DATA_BLOCK "Telegramindeling_rcv"
TITLE =
AUTHOR : DSB_TIM
FAMILY : Tim_rcv
NAME : Receive
VERSION : 0.1


  STRUCT
 Telegram101  :  STRUCT
besturing_remote  : BOOL ;
besturing_lokaal  : BOOL ;
pompen_blokkering  : BOOL ;
pompen_vrijgeven  : BOOL ;
niveaumeting1_voorkeuze  : BOOL ;
niveaumeting2_voorkeuze  : BOOL ;
regenpompen_blokkering  : BOOL ;
regenpompen_vrijgeven  : BOOL ;
END_STRUCT;
Telegram102  :  STRUCT
besturing_remote  : BOOL ;
besturing_lokaal  : BOOL ;
pompen_blokkering  : BOOL ;
pompen_vrijgeven  : BOOL ;
niveaumeting1_voorkeuze  : BOOL ;
niveaumeting2_voorkeuze  : BOOL ;
regenpompen_blokkering  : BOOL ;
regenpompen_vrijgeven  : BOOL ;
END_STRUCT;
Telegram103  :  STRUCT
besturing_remote  : BOOL ;
besturing_lokaal  : BOOL ;
pompen_blokkering  : BOOL ;
pompen_vrijgeven  : BOOL ;
niveaumeting1_voorkeuze  : BOOL ;
niveaumeting2_voorkeuze  : BOOL ;
regenpompen_blokkering  : BOOL ;
regenpompen_vrijgeven  : BOOL ;
END_STRUCT;
Telegram104  :  STRUCT
besturing_remote  : BOOL ;
besturing_lokaal  : BOOL ;
pompen_blokkering  : BOOL ;
pompen_vrijgeven  : BOOL ;
niveaumeting1_voorkeuze  : BOOL ;
niveaumeting2_voorkeuze  : BOOL ;
regenpompen_blokkering  : BOOL ;
regenpompen_vrijgeven  : BOOL ;
END_STRUCT;
Telegram105  :  STRUCT
besturing_remote  : BOOL ;
besturing_lokaal  : BOOL ;
pompen_blokkering  : BOOL ;
pompen_vrijgeven  : BOOL ;
niveaumeting1_voorkeuze  : BOOL ;
niveaumeting2_voorkeuze  : BOOL ;
regenpompen_blokkering  : BOOL ;
regenpompen_vrijgeven  : BOOL ;
END_STRUCT;
Telegram106  :  STRUCT
besturing_remote  : BOOL ;
besturing_lokaal  : BOOL ;
pompen_blokkering  : BOOL ;
pompen_vrijgeven  : BOOL ;
niveaumeting1_voorkeuze  : BOOL ;
niveaumeting2_voorkeuze  : BOOL ;
regenpompen_blokkering  : BOOL ;
regenpompen_vrijgeven  : BOOL ;
END_STRUCT;

Telegram140  :  STRUCT
reserve1  : WORD ;
END_STRUCT;
Telegram141  :  STRUCT
reserve2  : WORD ;
END_STRUCT;
Telegram142  :  STRUCT
reserve3  : WORD ;
END_STRUCT;
Telegram143  :  STRUCT
reserve4  : WORD ;
END_STRUCT;
Telegram144  :  STRUCT
reserve5  : WORD ;
END_STRUCT;
Telegram145  :  STRUCT
reserve6  : WORD ;
END_STRUCT;
Telegram146  :  STRUCT
laagwater  : WORD ;
END_STRUCT;
Telegram147  :  STRUCT
laagwater_herstel  : WORD ;
END_STRUCT;
Telegram148  :  STRUCT
hoogwater  : WORD ;
END_STRUCT;
Telegram149  :  STRUCT
hoogwater_herstel  : WORD ;
END_STRUCT;
Telegram150  :  STRUCT
dode_band_niveaumeting  : WORD ;
END_STRUCT;
Telegram151  :  STRUCT
reserve7  : WORD ;
END_STRUCT;
Telegram152  :  STRUCT
dode_band_logging  : WORD ;
END_STRUCT;
Telegram153  :  STRUCT
pomp_1_inslagpeil  : WORD ;
END_STRUCT;
Telegram154  :  STRUCT
pomp_2_inslagpeil  : WORD ;
END_STRUCT;
Telegram155  :  STRUCT
pomp_3_inslagpeil  : WORD ;
END_STRUCT;
Telegram156  :  STRUCT
pomp_4_inslagpeil  : WORD ;
END_STRUCT;
Telegram157  :  STRUCT
pomp_5_inslagpeil  : WORD ;
END_STRUCT;
Telegram158  :  STRUCT
pomp_6_inslagpeil  : WORD ;
END_STRUCT;
Telegram159  :  STRUCT
pomp_1_uitslagpeil  : WORD ;
END_STRUCT;
Telegram160  :  STRUCT
pomp_2_uitslagpeil  : WORD ;
END_STRUCT;
Telegram161  :  STRUCT
pomp_3_uitslagpeil  : WORD ;
END_STRUCT;
Telegram162  :  STRUCT
pomp_4_uitslagpeil  : WORD ;
END_STRUCT;
Telegram163  :  STRUCT
pomp_5_uitslagpeil  : WORD ;
END_STRUCT;
Telegram164  :  STRUCT
pomp_6_uitslagpeil  : WORD ;
END_STRUCT;
Telegram165  :  STRUCT
reserve8  : WORD ;
END_STRUCT;
Telegram166  :  STRUCT
reserve9  : WORD ;
END_STRUCT;
Telegram167  :  STRUCT
reserve10  : WORD ;
END_STRUCT;
Telegram168  :  STRUCT
reserve11  : WORD ;
END_STRUCT;
Telegram169  :  STRUCT
reserve12  : WORD ;
END_STRUCT;
Telegram170  :  STRUCT
reserve13  : WORD ;
END_STRUCT;
Telegram171  :  STRUCT
reserve14  : WORD ;
END_STRUCT;
Telegram172  :  STRUCT
reserve15  : WORD ;
END_STRUCT;


  END_STRUCT ;
BEGIN

Telegram101.besturing_remote   := FALSE;
Telegram101.besturing_lokaal   := FALSE;
Telegram101.pompen_blokkering   := FALSE;
Telegram101.pompen_vrijgeven   := FALSE;
Telegram101.niveaumeting1_voorkeuze   := FALSE;
Telegram101.niveaumeting2_voorkeuze   := FALSE;
Telegram101.regenpompen_blokkering   := FALSE;
Telegram101.regenpompen_vrijgeven   := FALSE;


Telegram102.besturing_remote   := FALSE;
Telegram102.besturing_lokaal   := FALSE;
Telegram102.pompen_blokkering   := FALSE;
Telegram102.pompen_vrijgeven   := FALSE;
Telegram102.niveaumeting1_voorkeuze   := FALSE;
Telegram102.niveaumeting2_voorkeuze   := FALSE;
Telegram102.regenpompen_blokkering   := FALSE;
Telegram102.regenpompen_vrijgeven   := FALSE;


Telegram103.besturing_remote   := FALSE;
Telegram103.besturing_lokaal   := FALSE;
Telegram103.pompen_blokkering   := FALSE;
Telegram103.pompen_vrijgeven   := FALSE;
Telegram103.niveaumeting1_voorkeuze   := FALSE;
Telegram103.niveaumeting2_voorkeuze   := FALSE;
Telegram103.regenpompen_blokkering   := FALSE;
Telegram103.regenpompen_vrijgeven   := FALSE;


Telegram104.besturing_remote   := FALSE;
Telegram104.besturing_lokaal   := FALSE;
Telegram104.pompen_blokkering   := FALSE;
Telegram104.pompen_vrijgeven   := FALSE;
Telegram104.niveaumeting1_voorkeuze   := FALSE;
Telegram104.niveaumeting2_voorkeuze   := FALSE;
Telegram104.regenpompen_blokkering   := FALSE;
Telegram104.regenpompen_vrijgeven   := FALSE;


Telegram105.besturing_remote   := FALSE;
Telegram105.besturing_lokaal   := FALSE;
Telegram105.pompen_blokkering   := FALSE;
Telegram105.pompen_vrijgeven   := FALSE;
Telegram105.niveaumeting1_voorkeuze   := FALSE;
Telegram105.niveaumeting2_voorkeuze   := FALSE;
Telegram105.regenpompen_blokkering   := FALSE;
Telegram105.regenpompen_vrijgeven   := FALSE;


Telegram106.besturing_remote   := FALSE;
Telegram106.besturing_lokaal   := FALSE;
Telegram106.pompen_blokkering   := FALSE;
Telegram106.pompen_vrijgeven   := FALSE;
Telegram106.niveaumeting1_voorkeuze   := FALSE;
Telegram106.niveaumeting2_voorkeuze   := FALSE;
Telegram106.regenpompen_blokkering   := FALSE;
Telegram106.regenpompen_vrijgeven   := FALSE;


Telegram140.reserve1 := W#16#0;
Telegram141.reserve2 := W#16#0;
Telegram142.reserve3 := W#16#0;
Telegram143.reserve4 := W#16#0;
Telegram144.reserve5 := W#16#0;
Telegram145.reserve6 := W#16#0;
Telegram146.laagwater := W#16#0;
Telegram147.laagwater_herstel := W#16#0;
Telegram148.hoogwater := W#16#0;
Telegram149.hoogwater_herstel := W#16#0;
Telegram150.dode_band_niveaumeting := W#16#0;
Telegram151.reserve7 := W#16#0;
Telegram152.dode_band_logging := W#16#0;
Telegram153.pomp_1_inslagpeil := W#16#0;
Telegram154.pomp_2_inslagpeil := W#16#0;
Telegram155.pomp_3_inslagpeil := W#16#0;
Telegram156.pomp_4_inslagpeil := W#16#0;
Telegram157.pomp_5_inslagpeil := W#16#0;
Telegram158.pomp_6_inslagpeil := W#16#0;
Telegram159.pomp_1_uitslagpeil := W#16#0;
Telegram160.pomp_2_uitslagpeil := W#16#0;
Telegram161.pomp_3_uitslagpeil := W#16#0;
Telegram162.pomp_4_uitslagpeil := W#16#0;
Telegram163.pomp_5_uitslagpeil := W#16#0;
Telegram164.pomp_6_uitslagpeil := W#16#0;
Telegram165.reserve8 := W#16#0;
Telegram166.reserve9 := W#16#0;
Telegram167.reserve10 := W#16#0;
Telegram168.reserve11 := W#16#0;
Telegram169.reserve12 := W#16#0;
Telegram170.reserve13 := W#16#0;
Telegram171.reserve14 := W#16#0;
Telegram172.reserve15 := W#16#0;



END_DATA_BLOCK

